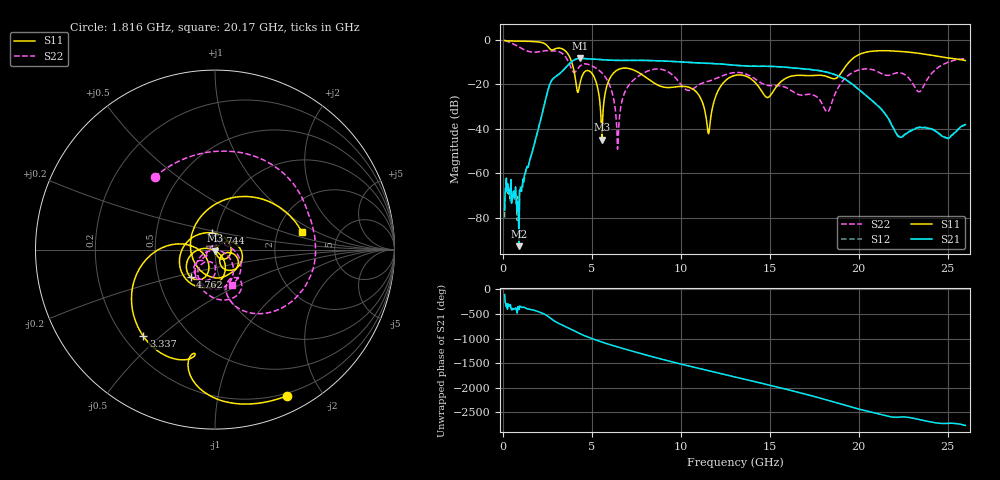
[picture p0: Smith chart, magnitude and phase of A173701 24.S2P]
!  2-Port S-parameters saved by WinCal
! VAR MeasName=S-Parameters (CALIBRATED_DATA) read from VNA (N5245A)
! VAR MeasDate=2017-6-7 10:29:58
! VAR NAME=A173701 24
! VAR FILENAME=A173701 24.S2P
! VAR DATE=2017-6-7 10:29:58
! VAR PHYS_PORTS=1,2
# Hz S DB R 50
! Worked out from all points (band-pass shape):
!   801 points, 100 MHz to 26 GHz, reference 50 ohm
!   highest |S21| = -8.34 dB at 4.341 GHz (marker M1); lowest = -92.7 dB at 909.4 MHz (marker M2)
!   |S21| within 3 dB of the highest: 3.665 GHz to 12.94 GHz (9.273 GHz wide, 112 % of centre)
!   lowest |S11| = -44.9 dB at 5.571 GHz (marker M3), VSWR 1.01, Z = 50 - j0.568 ohm
!   |S11| at or under -10 dB: 3.87 GHz to 19.46 GHz (15.59 GHz wide, 134 % of centre)
!   |S22| runs from -49.1 to -0.3 dB; largest |S21 - S12| = 0.004
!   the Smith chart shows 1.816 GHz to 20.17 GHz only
!   S11 on the Smith chart (normalised r, x): 1.816 GHz: 0.17, -1.60; 3.337 GHz: 0.28, -0.44; 4.762 GHz: 0.73, -0.23; 8.744 GHz: 0.95, +0.18; 20.17 GHz: 2.74, +0.72
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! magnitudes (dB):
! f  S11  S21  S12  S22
! 100 MHz  -0.3  -76.7  -79.9  -0.3
! 909.4 MHz  -0.6  -92.7  -86.1  -3.2
! 1.816 GHz  -0.8  -45.5  -45.3  -5.6
! 2.658 GHz  -4.2  -19.7  -19.6  -5.0
! 3.337 GHz  -4.1  -14.1  -14.1  -6.1
! 4.341 GHz  -19.4  -8.3  -8.3  -11.8
! 4.438 GHz  -16.6  -8.3  -8.3  -11.2
! 4.762 GHz  -13.8  -8.5  -8.5  -10.9
! 5.571 GHz  -44.9  -8.9  -8.9  -14.9
! 6.478 GHz  -13.4  -9.3  -9.2  -46.7
! 7.061 GHz  -12.8  -9.2  -9.2  -20.6
! 8.744 GHz  -20.5  -9.4  -9.5  -13.1
! 10.75 GHz  -22.5  -10.3  -10.3  -21.7
! 11.56 GHz  -42.3  -10.6  -10.6  -18.6
! 13.05 GHz  -16.0  -11.4  -11.4  -14.7
! 14.86 GHz  -25.9  -11.9  -11.9  -20.5
! 17.39 GHz  -16.1  -13.5  -13.4  -24.7
! 18.26 GHz  -16.6  -14.7  -14.6  -32.4
! 20.17 GHz  -6.1  -23.4  -23.4  -13.3
! 21.69 GHz  -4.9  -35.8  -35.6  -15.9
! 23.41 GHz  -6.1  -39.4  -39.2  -23.4
! 26 GHz  -9.3  -38.1  -38.0  -8.6
